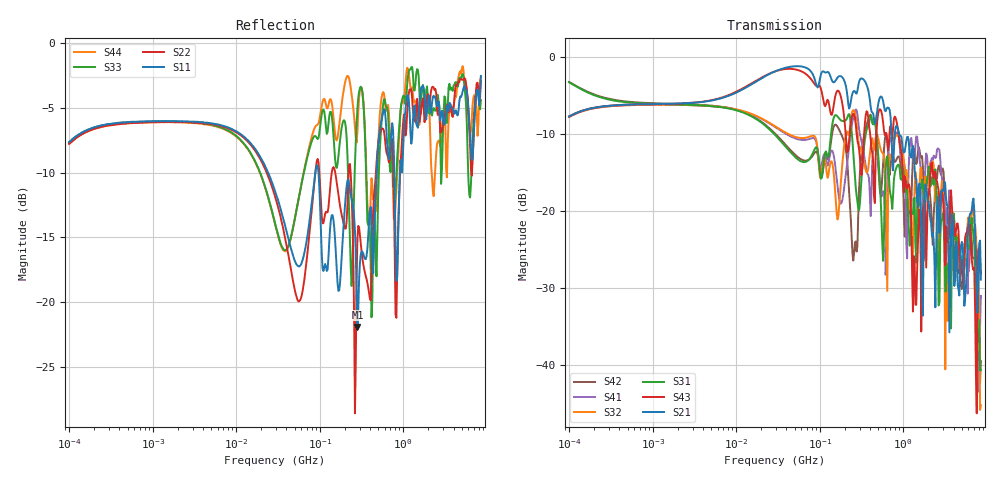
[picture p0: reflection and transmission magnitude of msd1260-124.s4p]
# MHz S MA R 50
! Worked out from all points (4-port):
!   498 points, 100 kHz to 8.5 GHz, reference 50 ohm
!   strongest paths, dB at 100 kHz, 1.698 MHz, 29.49 MHz, 500.7 MHz, 8.5 GHz:
!     S21: -7.7, -6.1, -1.8, -6.2, -28.9
!     S43: -7.7, -6.1, -1.9, -7.4, -28.3
!     S31: -3.3, -6.1, -10.2, -12.6, -40.7
!     S32: -7.8, -6.2, -9.0, -10.5, -45.2
!     S41: -7.8, -6.2, -9.1, -13.2, -31.0
!     S42: -3.2, -6.1, -10.0, -13.9, -39.5
!   lowest |S11| = -21.9 dB at 282.9 MHz (marker M1), VSWR 1.17, Z = 57 - j4.93 ohm
!   |S11| at or under -10 dB: 24.13 MHz to 88.79 MHz (64.65 MHz wide, 115 % of centre); 96.74 MHz to 480.7 MHz (384 MHz wide, 133 % of centre); 780.6 MHz to 911.4 MHz (130.8 MHz wide, 15.5 % of centre)
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0.1  0.415 32.7  0.4108 33.3  0.6845 -19.5  0.4078 -147.3
     0.4108 33.3  0.4085 32.7  0.4085 -147.2  0.6888 -19.2
     0.6845 -19.5  0.4085 -147.2  0.4146 32.8  0.4109 33.2
     0.4078 -147.3  0.6888 -19.2  0.4109 33.2  0.4094 32.7
282.8688  0.08022 -32.4  0.6041 -43.3  0.1147 -133.2  0.4224 4.3
          0.6041 -43.3  0.1753 21.1  0.3265 -26.5  0.05911 -146.2
          0.1147 -133.2  0.3265 -26.5  0.5606 0.8  0.2863 -78.0
          0.4224 4.3  0.05911 -146.2  0.2863 -78.0  0.4582 -28.5
1498.389  0.4717 -129.5  0.1055 159.3  0.1125 -130.8  0.2722 -167.7
          0.1055 159.3  0.5644 -147.2  0.06294 -157.6  0.2409 -142.6
          0.1125 -130.8  0.06294 -157.6  0.7896 -151.2  0.0618 -68.9
          0.2722 -167.7  0.2409 -142.6  0.0618 -68.9  0.5093 -158.9
3651.237  0.5837 9.5  0.03385 26.5  0.0362 -6.8  0.1103 -90.8
          0.03385 26.5  0.5815 -2.1  0.08925 17.7  0.05337 -74.9
          0.0362 -6.8  0.08925 17.7  0.662 0.2  0.1174 -37.3
          0.1103 -90.8  0.05337 -74.9  0.1174 -37.3  0.5419 14.6
5898.28  0.6157 -126.1  0.06454 115.6  0.05999 159.8  0.02901 -171.4
         0.06454 115.6  0.6052 -139.9  0.08222 -168.3  0.04307 151.0
         0.05999 159.8  0.08222 -168.3  0.374 -169.0  0.07801 66.0
         0.02901 -171.4  0.04307 151.0  0.07801 66.0  0.6135 -155.8
6920.76  0.4104 68.5  0.1204 -13.6  0.06762 21.6  0.07596 57.6
         0.1204 -13.6  0.4246 31.5  0.09627 39.4  0.04937 30.9
         0.06762 21.6  0.09627 39.4  0.4928 10.8  0.04131 -32.2
         0.07596 57.6  0.04937 30.9  0.04131 -32.2  0.6168 9.0
8500  0.7477 -31.8  0.03579 -131.2  0.00927 2.7  0.02807 -53.8
      0.03579 -131.2  0.7147 -40.1  0.005474 18.9  0.01058 -74.2
      0.00927 2.7  0.005474 18.9  0.6028 -39.4  0.03863 -117.5
      0.02807 -53.8  0.01058 -74.2  0.03863 -117.5  0.7384 -47.2
